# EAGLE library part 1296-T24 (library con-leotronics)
1.27mm SINGLE ROW FEMALE SOCKET Source: http://www.leotronics.co.uk/Conexcon/Data%20Sheets/sec.%20A/1296ing.pdf
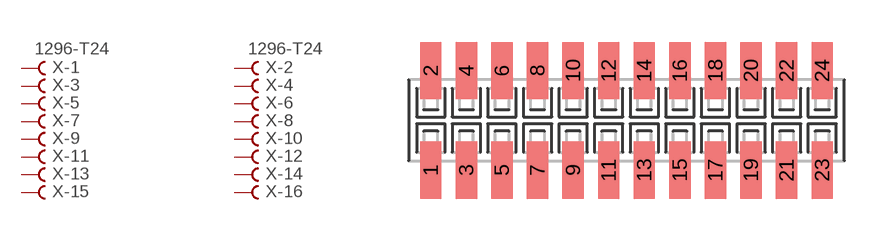
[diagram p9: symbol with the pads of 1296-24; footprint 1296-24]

Designator prefix X; gates -1=FVAL -2=FVAL -3=F -4=F -5=F -6=F -7=F -8=F -9=F -10=F -11=F -12=F -13=F -14=F -15=F -16=F -17=F -18=F -19=F -20=F -21=F -22=F -23=F -24=F

## 1296-T24 (OC_FARNELL: unknown; OC_NEWARK: unknown)  [1296-24]
1  -1:B  pas
2  -2:B  pas
3  -3:B  pas
4  -4:B  pas
5  -5:B  pas
6  -6:B  pas
7  -7:B  pas
8  -8:B  pas
9  -9:B  pas
10  -10:B  pas
11  -11:B  pas
12  -12:B  pas
13  -13:B  pas
14  -14:B  pas
15  -15:B  pas
16  -16:B  pas
17  -17:B  pas
18  -18:B  pas
19  -19:B  pas
20  -20:B  pas
21  -21:B  pas
22  -22:B  pas
23  -23:B  pas
24  -24:B  pas

## Footprint 1296-24 (pad centres in mm)
1.27mm SINGLE ROW FEMALE SOCKET Source: http://www.leotronics.co.uk/Conexcon/Data%20Sheets/sec.%20A/1296ing.pdf
smd 0.76 x 2.05: 1 -6.985,-1.78; 2 -6.985,1.78; 3 -5.715,-1.78; 4 -5.715,1.78; 5 -4.445,-1.78; 6 -4.445,1.78; 7 -3.175,-1.78; 8 -3.175,1.78; 9 -1.905,-1.78; 10 -1.905,1.78; 11 -0.635,-1.78; 12 -0.635,1.78; 13 0.635,-1.78; 14 0.635,1.78; 15 1.905,-1.78; 16 1.905,1.78; 17 3.175,-1.78; 18 3.175,1.78; 19 4.445,-1.78; 20 4.445,1.78; 21 5.715,-1.78; 22 5.715,1.78; 23 6.985,-1.78; 24 6.985,1.78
